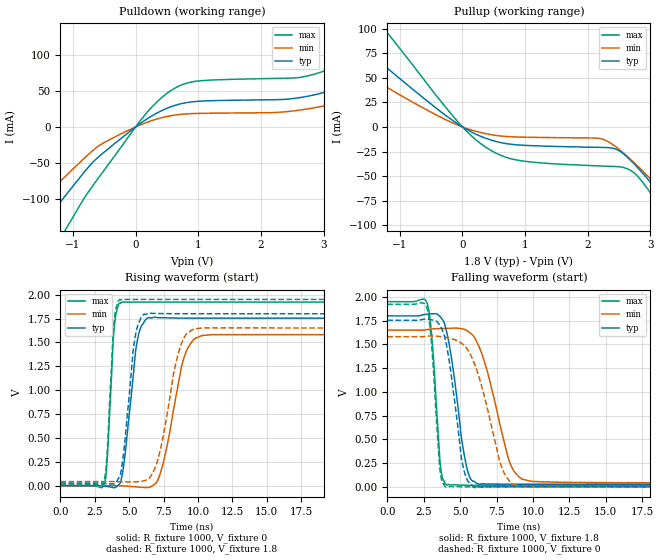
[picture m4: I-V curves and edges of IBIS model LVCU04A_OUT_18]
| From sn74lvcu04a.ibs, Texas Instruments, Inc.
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[Model]   LVCU04A_OUT_18
Model_type  Output
Vref =   0
Rref =   1000
Cref =   30p
Vmeas =   0.9
| variable   typ   min   max
C_comp   8.28pF   4.11pF   14.74pF
| C_pullup   6.96pF   4.11pF   8.25pF
| C_pulldown   9.60pF   4.63pF   14.74pF
[Temperature Range]   40   100   -40
| Ambient temperature   25   85   -40
[Voltage range]   1.8   1.65   1.95
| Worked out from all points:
|   slope of the pulldown table from 0 to 0.27 V, typ, clamps not added: 17.1 ohm
|   slope of the pullup table from 0 to 0.27 V, typ, clamps not added: 29.9 ohm
|   rising waveform, R_fixture 1000, V_fixture 0: 20-80 % time 743ps typ, 1.23ns min, 400ps max; typ from 0 V to 1.75 V
|   falling waveform, R_fixture 1000, V_fixture 1.8: 20-80 % time 919ps typ, 1.56ns min, 495ps max; typ from 1.8 V to 0.027 V
|   rising waveform, R_fixture 1000, V_fixture 1.8: 20-80 % time 687ps typ, 1.23ns min, 399ps max; typ from 0.027 V to 1.8 V
|   falling waveform, R_fixture 1000, V_fixture 0: 20-80 % time 880ps typ, 1.58ns min, 497ps max; typ from 1.75 V to 0 V
[Pulldown]
| LVCU04A_OUT_18
|   Voltage   I(typ)   I(min)   I(max)
-5.5V     -562.8mA   -456mA     -714.6mA
-1.87V    -176.7mA   -133mA     -245.9mA
-1.485V   -135.1mA   -99.63mA   -194.2mA
-1.07V    -89.57mA   -64.08mA   -135.1mA
-570mV    -39.87mA   -25.16mA   -67.84mA
70mV      4.491mA    2.617mA    8.125mA
615mV     29.45mA    16.27mA    53.12mA
2.815V    43.69mA    25.92mA    72.1mA
4.325V    93.52mA    64.21mA    142.7mA
5.155V    134.5mA    96.03mA    199.6mA
6.155V    191.3mA    141.3mA    276.1mA
11V       510.2mA    405.2mA    689.3mA
[Pullup]
| LVCU04A_OUT_18
|   Voltage   I(typ)   I(min)   I(max)
-5.5V     324.9mA    249.5mA    454.8mA
-2.68V    143.9mA    103mA      216.3mA
-2.015V   104.9mA    73.15mA    161.8mA
-1.32V    66.21mA    44.72mA    105.6mA
360mV     -11.3mA    -6.711mA   -20.18mA
980mV     -18.71mA   -10.42mA   -34.85mA
2.465V    -23.03mA   -21.11mA   -40.36mA
2.81V     -42.39mA   -40.68mA   -51.19mA
3.355V    -85.4mA    -77.55mA   -102.6mA
3.555V    -102.9mA   -92.26mA   -124.5mA
3.77V     -122.5mA   -108.6mA   -148.9mA
11V       -881.1mA   -746.6mA   -1.074A
[Ramp]
| LVCU04A_OUT_18
| variable   typ   min   max
dV/dt_r   1.07/8.18E-10   0.96/1.27E-09   1.17/4.45E-10
dV/dt_f   1.08/1.01E-09   0.98/1.60E-09   1.18/5.10E-10
R_load = 1000
[Rising Waveform]
| LVCU04A_OUT_18
R_fixture =   1000
C_fixture =   0
L_fixture =   0
V_fixture =   0
V_fixture_min = 0
V_fixture_max = 0
|   Time   V(typ)   V(min)   V(max)
0s        194.2pV    4.892nV    16.26pV
3.21ns    -4.905mV   228uV      33.07mV
3.88ns    -21.51mV   164.7uV    1.602V
4.3ns     19.8mV     -1.165mV   1.913V
5.53ns    1.471V     -13.08mV   1.922V
6.325ns   1.756V     -20.14mV   1.922V
7.27ns    1.759V     133.2mV    1.922V
8.835ns   1.755V     1.265V     1.922V
9.815ns   1.754V     1.544V     1.922V
24.99ns   1.754V     1.581V     1.922V
[Falling Waveform]
| LVCU04A_OUT_18
R_fixture =   1000
C_fixture =   0
L_fixture =   0
V_fixture =   1.8
V_fixture_min = 1.65
V_fixture_max = 1.95
|   Time   V(typ)   V(min)   V(max)
0s        1.8V       1.65V      1.95V
2.75ns    1.818V     1.656V     1.925V
3.09ns    1.822V     1.662V     1.517V
3.63ns    1.792V     1.666V     251.2mV
4.055ns   1.643V     1.669V     20.05mV
5.36ns    274.1mV    1.654V     16.62mV
6.155ns   35.22mV    1.524V     15.95mV
8.31ns    28.09mV    298.6mV    16.26mV
9.25ns    27.47mV    82.03mV    16.27mV
24.99ns   27.13mV    42.43mV    16.27mV
[Rising Waveform]
| LVCU04A_OUT_18
R_fixture =   1000
C_fixture =   0
L_fixture =   0
V_fixture =   1.8
V_fixture_min = 1.65
V_fixture_max = 1.95
|   Time   V(typ)   V(min)   V(max)
0s        27.13mV    42.42mV    16.27mV
3.135ns   23.98mV    42.55mV    40.65mV
3.375ns   20.62mV    42.53mV    302.7mV
3.87ns    17.81mV    42.35mV    1.673V
4.285ns   94.27mV    41.48mV    1.948V
5.365ns   1.5V       39.26mV    1.95V
6.045ns   1.793V     50.28mV    1.95V
6.995ns   1.803V     229.7mV    1.95V
9.58ns    1.8V       1.632V     1.95V
24.99ns   1.8V       1.65V      1.95V
[Falling Waveform]
| LVCU04A_OUT_18
R_fixture =   1000
C_fixture =   0
L_fixture =   0
V_fixture =   0
V_fixture_min = 0
V_fixture_max = 0
|   Time   V(typ)   V(min)   V(max)
0s        1.754V     1.581V     1.922V
2.715ns   1.765V     1.585V     1.884V
3.055ns   1.758V     1.589V     1.467V
3.59ns    1.704V     1.583V     216.7mV
4ns       1.539V     1.573V     352.2uV
5.13ns    266.3mV    1.508V     532.1uV
5.965ns   -7.347mV   1.306V     -317.6uV
7.75ns    542.7uV    252.9mV    -22.98uV
8.695ns   245.6uV    21.32mV    -1.087uV
24.99ns   8.87nV     1.146uV    14.19nV
